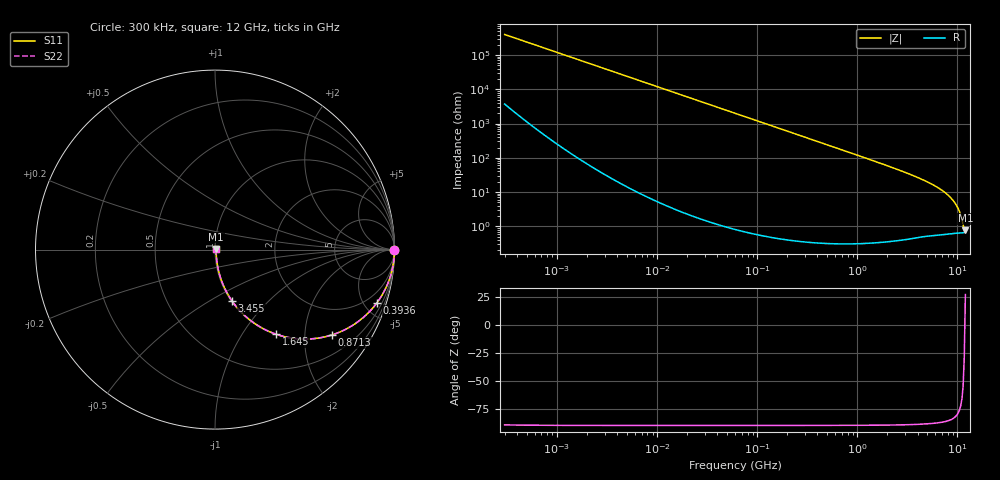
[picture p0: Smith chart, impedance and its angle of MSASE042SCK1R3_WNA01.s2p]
! MSASE042SCK1R3_WNA01  S-PARAMETER MODEL  ( General Type )
! Model Generated by TAIYO YUDEN Corporation (http://www.ty-top.com)
! Version 1.0
! TAIYO YUDEN Control No. 120810
! Copyright(c) 2012 TAIYO YUDEN CO.,LTD. All Rights Reserved.
! Product Description (link to TY-COMPAS)
! https://ds.yuden.co.jp/TYCOMPAS/or/detail?pn=MSASE042SCK1R3AWNA01&u=M
! Products Name : Multilayer Ceramic Capacitors
! Characteristics :
!  Capacitance : 1.3 pF , Rated Voltage : 16V , TCC : CK / C0K
!  Case Size : 0.4 x 0.2 / 0.016 x 0.008 [mm/inch] , Thickness : 0.2 / 0.008 [mm/inch]
!  (Conditions: Temperature = 25 degC , DC Bias Current/Voltage = 0A / 0V)
! External Node Assignments :
!  1  o---| |---o  2
! GND o---------o GND
! Frequency Range : 0.3MHz  -  12000MHz  [ 401 STEP ]
# MHz S RI R 50
! Freq[MHz].  S11 Real  S11 Imag  S21 Real  S21 Imag  S12 Real  S12 Imag  S22 Real  S22 Imag
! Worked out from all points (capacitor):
!   401 points, 300 kHz to 12 GHz, reference 50 ohm
!   read as one part in series: C = 1.32 pF near 316.3 kHz
!   lowest |Z| = 756 mohm at 12 GHz (marker M1)
!   series resonance near 11.85 GHz, so ESL is about 140 pH
!   S11 on the Smith chart (normalised r, x): 300 kHz: open; 393.6 MHz: 1.01, -6.10; 871.3 MHz: 1.01, -2.74; 1.645 GHz: 1.01, -1.43; 3.455 GHz: 1.01, -0.64; 12 GHz: 1.01, +0.01
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0.3  1 -0.00025  2.38e-06 0.00025  2.38e-06 0.00025  1 -0.00025
1.769972  1 -0.00147  3.96e-06 0.00147  3.96e-06 0.00147  1 -0.00147
10.44266  0.9999 -0.00869  7.92e-05 0.00869  7.92e-05 0.00869  0.9999 -0.00869
60  0.9975 -0.0498  0.0025 0.0498  0.0025 0.0498  0.9975 -0.0498
155.7172  0.9834 -0.1274  0.0166 0.1274  0.0166 0.1274  0.9834 -0.1274
353.9943  0.9199 -0.271  0.0801 0.271  0.0801 0.271  0.9199 -0.271
393.5654  0.9028 -0.2957  0.0972 0.2957  0.0972 0.2957  0.9028 -0.2957
585.5907  0.8071 -0.3938  0.1929 0.3938  0.1929 0.3938  0.8071 -0.3938
871.3074  0.6529 -0.4749  0.3471 0.4749  0.3471 0.4749  0.6529 -0.4749
1197.383  0.497 -0.4984  0.503 0.4984  0.503 0.4984  0.497 -0.4984
1645.489  0.3401 -0.4714  0.6599 0.4714  0.6599 0.4714  0.3401 -0.4714
2088.533  0.2388 -0.4232  0.7612 0.4232  0.7612 0.4232  0.2388 -0.4232
3454.93  0.0954 -0.2871  0.9046 0.2871  0.9046 0.2871  0.0954 -0.2871
4623.766  0.0508 -0.2086  0.9492 0.2086  0.9492 0.2086  0.0508 -0.2086
5868.704  0.0285 -0.1499  0.9715 0.1499  0.9715 0.1499  0.0285 -0.1499
7064.448  0.0175 -0.1078  0.9825 0.1078  0.9825 0.1078  0.0175 -0.1078
8281.503  0.0114 -0.0738  0.9886 0.0738  0.9886 0.0738  0.0114 -0.0738
9207.246  0.00886 -0.0518  0.9911 0.0518  0.9911 0.0518  0.00886 -0.0518
9968.853  0.00755 -0.0357  0.9924 0.0357  0.9924 0.0357  0.00755 -0.0357
10511.28  0.00698 -0.025  0.993 0.025  0.993 0.025  0.00698 -0.025
11380.75  0.00649 -0.00916  0.9935 0.00916  0.9935 0.00916  0.00649 -0.00916
12000  0.00671 0.00337  0.9933 -0.00337  0.9933 -0.00337  0.00671 0.00337
